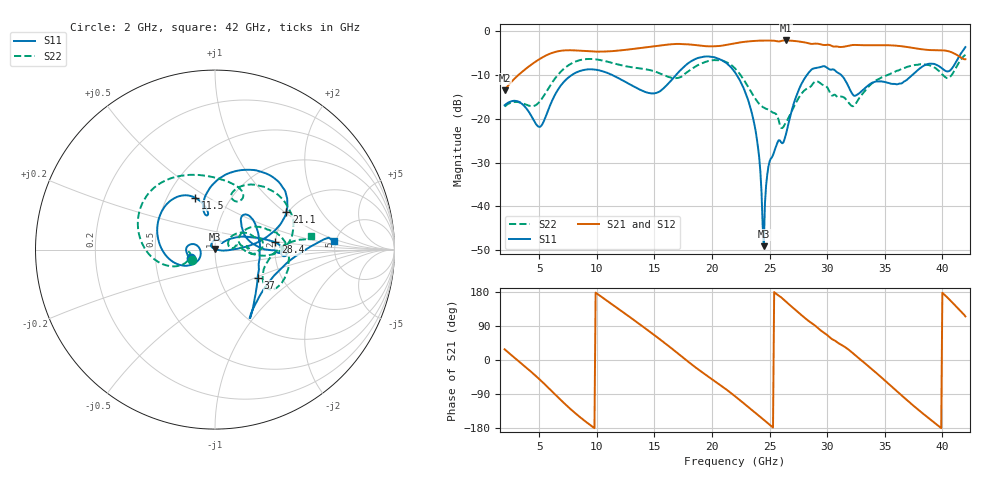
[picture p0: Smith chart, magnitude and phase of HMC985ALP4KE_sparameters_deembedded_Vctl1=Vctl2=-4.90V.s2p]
!s2p File: Measurements: S11, S21, S12, S22
# GHz S dB R 50.0
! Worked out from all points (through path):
!   401 points, 2 GHz to 42 GHz, reference 50 ohm
!   highest |S21| = -2.06 dB at 26.4 GHz (marker M1); lowest = -13.4 dB at 2 GHz (marker M2)
!   lowest |S11| = -49.1 dB at 24.5 GHz (marker M3), VSWR 1.01, Z = 49.9 + j0.329 ohm
!   |S11| at or under -10 dB: start of sweep to 7.813 GHz; 22.16 GHz to 28.24 GHz (6.078 GHz wide, 24.1 % of centre); 31.23 GHz to 37.37 GHz (6.143 GHz wide, 17.9 % of centre)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
!   |S22| runs from -22.1 to -5.3 dB; largest |S21 - S12| = 0.00085
!   S11 on the Smith chart (normalised r, x): 2 GHz: 0.76, -0.07; 11.5 GHz: 0.68, +0.44; 21.1 GHz: 1.97, +1.02; 28.4 GHz: 2.00, +0.18; 37 GHz: 1.52, -0.52; 42 GHz: 4.79, +0.79
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2  -16.87 -161.7  -13.43 28.3  -13.43 28.3  -17.17 -155.5
5  -21.82 -172.5  -6.37 -50.1  -6.37 -50.1  -16.17 -159.8
6.3  -14.85 -150.3  -4.75 -88.3  -4.76 -88.3  -11.02 -161.6
8.7  -8.92 150.4  -4.44 -154.6  -4.44 -154.6  -6.46 151.3
11.5  -10.16 111.1  -4.47 143.1  -4.47 143.1  -7.31 105.1
13.6  -13.12 101.2  -3.85 97.2  -3.85 97.2  -8.40 75.6
15.4  -13.81 105.8  -3.25 56.5  -3.25 56.5  -9.50 62.0
17.9  -7.33 80.3  -2.94 -3.5  -2.94 -3.5  -9.20 72.0
21.1  -6.96 27.6  -3.14 -74.4  -3.14 -74.3  -6.86 16.0
22  -9.35 17.0  -2.71 -95.5  -2.71 -95.5  -8.45 0.6
23.6  -20.21 0.0  -2.17 -135.2  -2.17 -135.2  -14.72 -4.5
24.5  -49.12 109.4  -2.08 -157.9  -2.07 -157.9  -17.41 8.0
25  -29.73 132.3  -2.10 -170.6  -2.10 -170.6  -18.00 10.9
26.4  -23.73 41.5  -2.06 154.7  -2.06 154.7  -20.95 32.7
28.4  -9.42 6.9  -2.71 102.7  -2.71 102.7  -12.86 18.2
28.7  -8.59 2.0  -2.85 96.5  -2.85 96.5  -12.18 16.3
30.7  -8.95 -3.1  -3.44 50.6  -3.44 50.6  -14.50 2.0
32.5  -14.63 31.4  -3.09 10.9  -3.09 10.9  -16.45 27.4
35.4  -11.82 19.3  -3.16 -64.6  -3.16 -64.6  -9.79 19.4
37  -10.88 -33.7  -3.57 -107.7  -3.58 -107.7  -8.06 5.0
39.8  -8.09 -57.6  -4.29 -177.2  -4.28 -177.2  -9.27 -36.0
42  -3.58 4.0  -6.34 115.0  -6.35 115.1  -5.33 8.3
